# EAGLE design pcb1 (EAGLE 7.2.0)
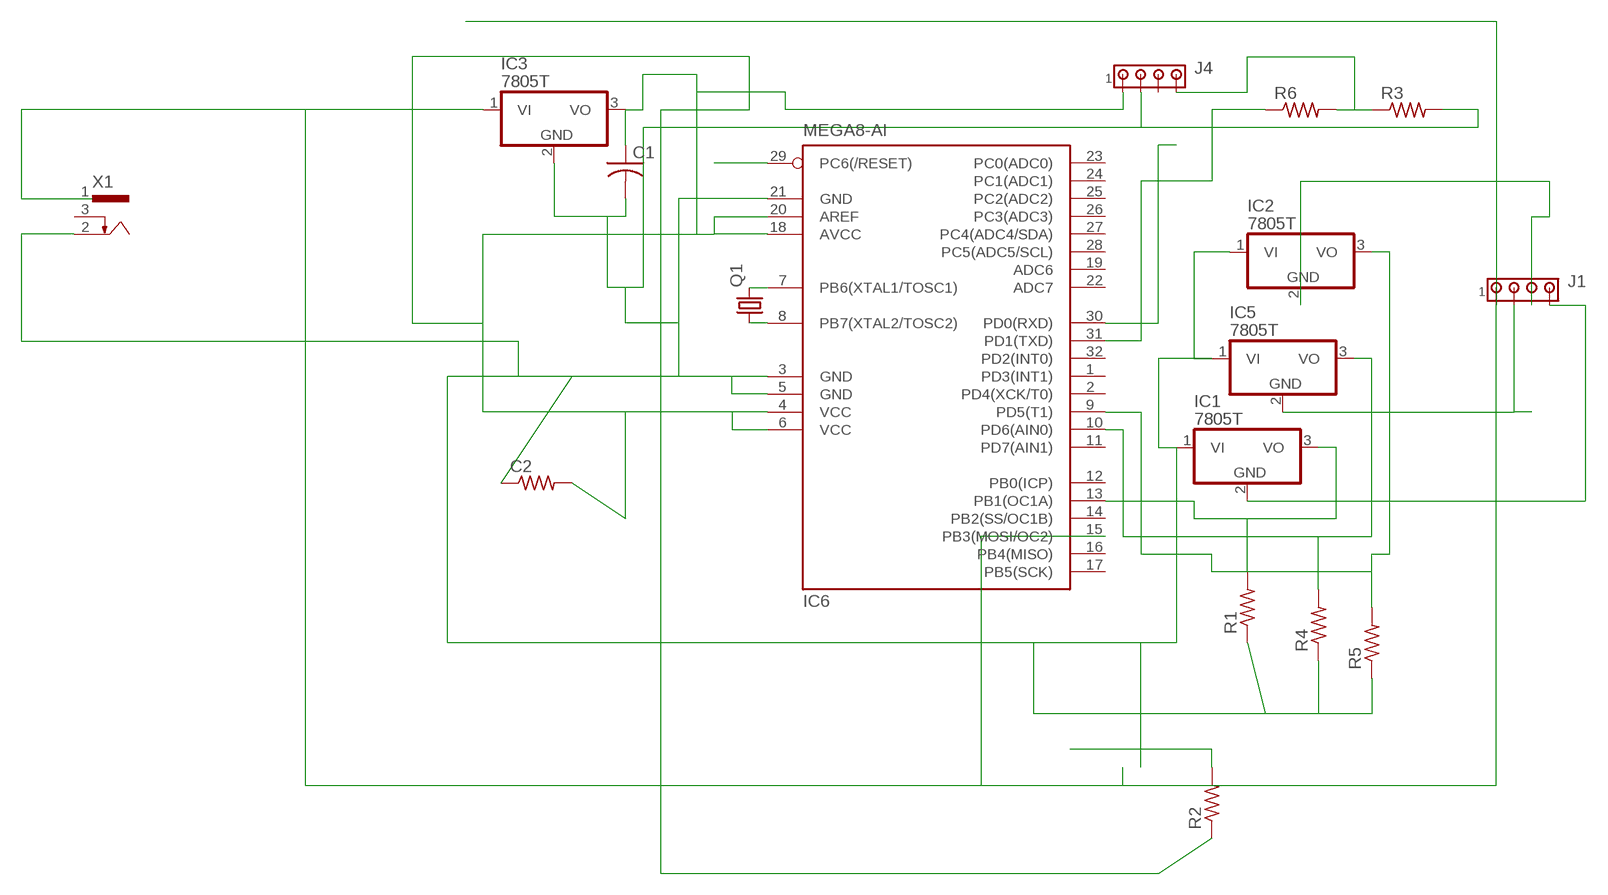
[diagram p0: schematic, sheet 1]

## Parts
C1  C-US025-025X050  [C025-025X050]
C2  R-US_M1206  [M1206]
IC1  7805T  [TO220H]
IC2  7805T  [TO220H]
IC3  7805T  [TO220H]
IC5  7805T  [TO220H]
IC6  MEGA8-AI  [TQFP32-08]
J1  MTA04-100  [10X04MTA]
J4  MTA04-100  [10X04MTA]
Q1  CRYSTALHC49S  [HC49/S]
R1  R-US_M1206  [M1206]
R2  R-US_M1206  [M1206]
R3  R-US_M1206  [M1206]
R4  R-US_M1206  [M1206]
R5  R-US_M1206  [M1206]
R6  R-US_M1206  [M1206]
X1  733980-62  [733980-62]

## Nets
N$1: IC6.7(PB6(XTAL1/TOSC1)) Q1.2
N$2: IC6.8(PB7(XTAL2/TOSC2)) Q1.1
N$5: IC2.2(GND) J1.3
N$6: IC1.3(VO) IC6.13(PB1(OC1A)) R1.2
N$7: IC6.15(PB3(MOSI/OC2))
N$8: IC5.3(VO) IC6.10(PD6(AIN0)) R4.2
N$9: R2.2
N$10: IC2.3(VO) IC6.9(PD5(T1)) R5.2
N$11: C1.2 C2.1 IC1.1(VI) IC2.1(VI) IC3.2(GND) IC5.1(VI) IC6.3(GND) IC6.5(GND) IC6.21(GND) J4.2 R1.1 R3.2 R4.1 R5.1 X1.2
N$12: IC5.2(GND) J1.2
N$13: IC1.2(GND) J1.4
N$14: IC6.29(PC6(/RESET))
N$15: IC6.30(PD0(RXD))
N$18: IC6.31(PD1(TXD)) R6.1
N$20: J4.4 R3.1 R6.2
N$23: IC3.1(VI) J1.1 X1.1
N$24: C1.1 C2.2 IC3.3(VO) IC6.4(VCC) IC6.6(VCC) IC6.18(AVCC) IC6.20(AREF) J4.1 R2.1
Unconnected: IC6.1(PD3(INT1)) IC6.2(PD4(XCK/T0)) IC6.11(PD7(AIN1)) IC6.12(PB0(ICP)) IC6.14(PB2(SS/OC1B)) IC6.16(PB4(MISO)) IC6.17(PB5(SCK)) IC6.19(ADC6) IC6.22(ADC7) IC6.23(PC0(ADC0)) IC6.24(PC1(ADC1)) IC6.25(PC2(ADC2)) IC6.26(PC3(ADC3)) IC6.27(PC4(ADC4/SDA)) IC6.28(PC5(ADC5/SCL)) IC6.32(PD2(INT0)) J4.3 X1.3

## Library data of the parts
C1 = adafruit:C-US: CAPACITOR, American symbol
C2 R1-R6 = adafruit:R-US_: RESISTOR, American symbol
IC1-IC3 IC5 = adafruit:78*: Positive VOLTAGE REGULATOR Added bigger pads to the TO-92 package
IC6 = atmel:MEGA8: MICROCONTROLLER 8 Kbytes FLASH, 1 kbytes SRAM, 512 bytes EEPROM, USART, 6-channel 10 bit ADC, 2-channel 8 bit ADC Pin compatible with Atmega48, ATMega88, ATMega168 Source: avr.lbr; MPN: ATMEGA8-16AU; OC_FARNELL: 9171371; OC_NEWARK: 73M8863
J1 J4 = con-amp:MTA04-100: AMP connector
Q1 = adafruit:CRYSTAL: CRYSTAL; OC_FARNELL: 1667008; OC_NEWARK: unknown
X1 = con-conrad:73398?: FEMALE PRINT CONNECTOR Niedervolt-Steckverbinder Distributor Conrad

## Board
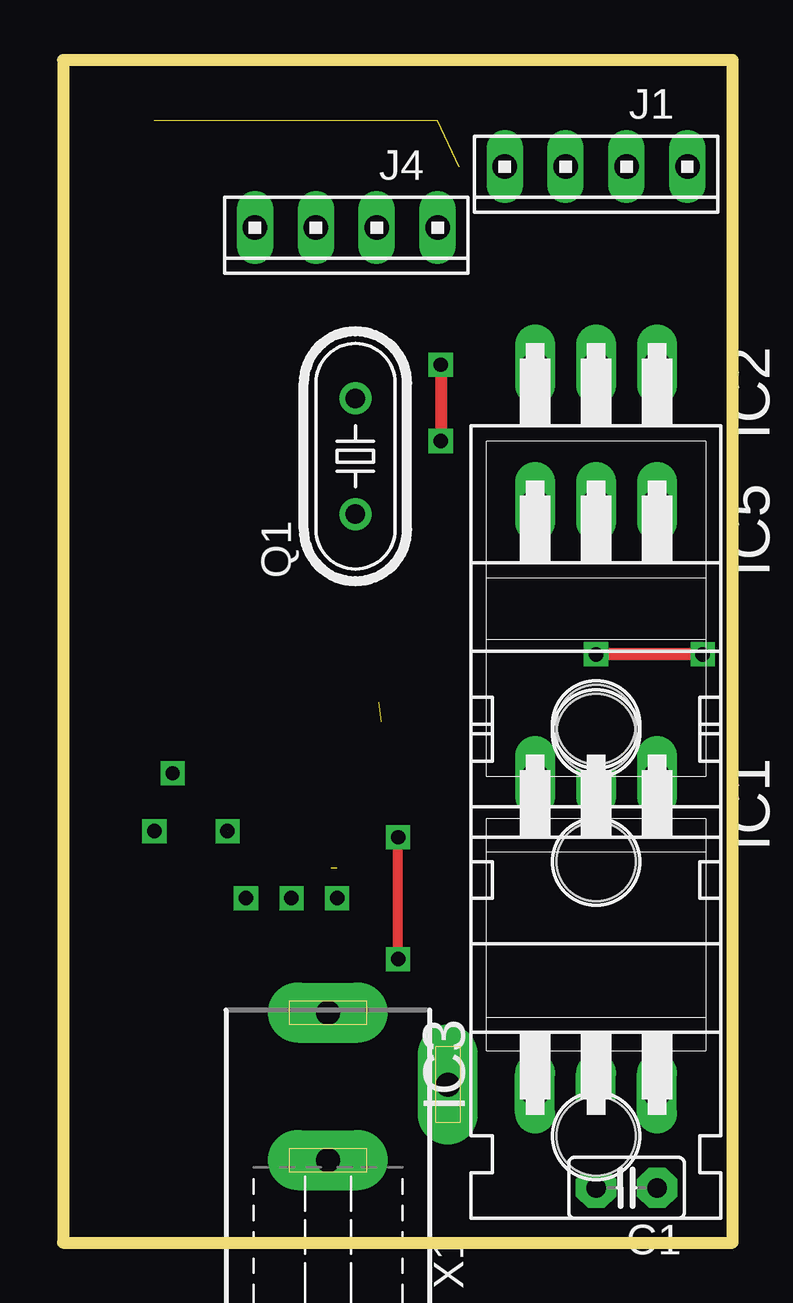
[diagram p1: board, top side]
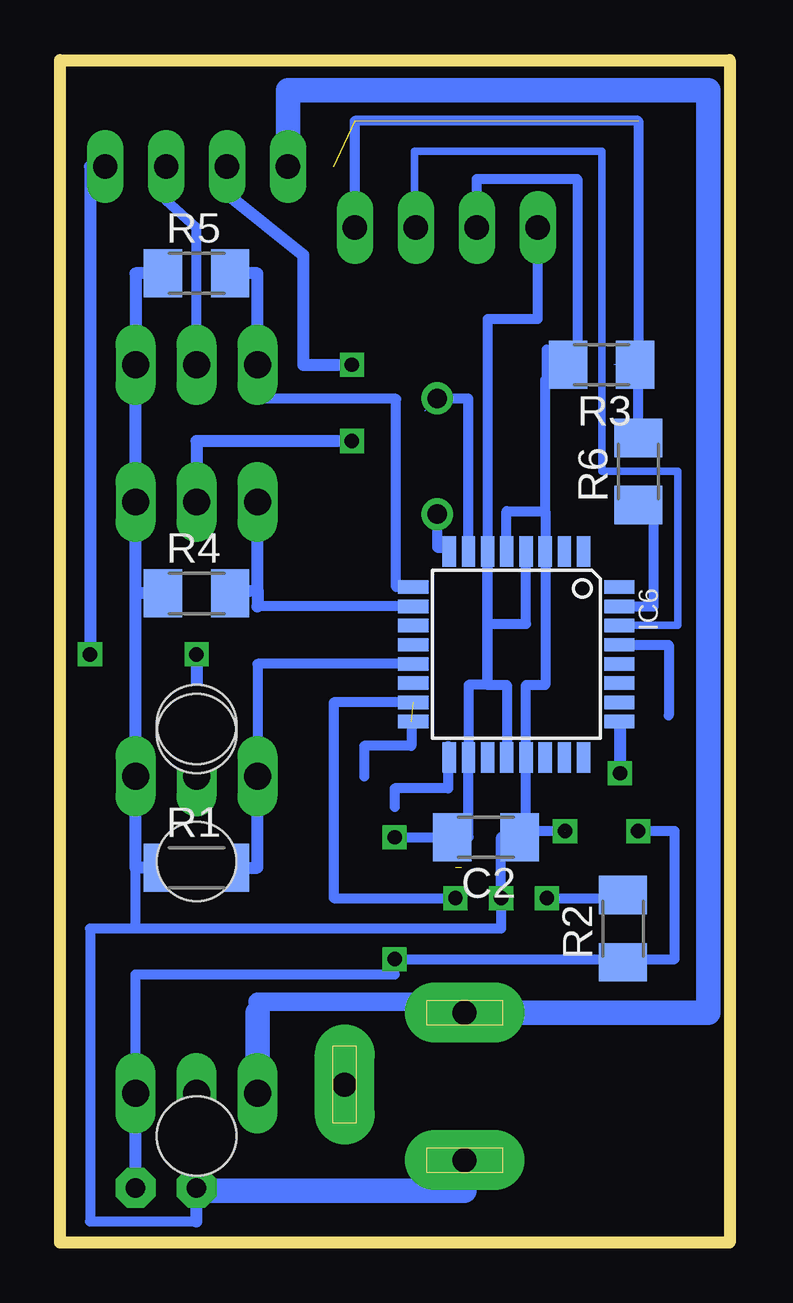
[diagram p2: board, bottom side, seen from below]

Size 27.92 x 49.28 mm. Coordinates in mm from the lower left corner, seen from the top.
Outline: 0,0 27.92,0 27.92,49.28 0,49.28 0,0
Copper layers (1*16): Top 0.035mm / dielectric 1.5mm / Bottom 0.035mm
Design rules "default": minimum track width 10mil, minimum drill 24mil, track to track 8mil, track to pad 8mil, pad to pad 8mil, via to via 8mil, smd to smd 8mil, copper to edge 40mil, drill to drill 8mil, minimum pad ring 10mil, minimum via ring 8mil, stop-mask expansion 4mil, vias tented up to drill 0mil, thermal gap 10mil

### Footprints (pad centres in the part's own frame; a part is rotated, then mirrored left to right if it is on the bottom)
C025-025X050 = drill 0.813 pad 1.676 octagon: 1 -1.27,0; 2 1.27,0
M1206 = smd 1.6 x 2: 1 -1.4,0; 2 1.4,0
TO220H = drill 1.118 long: 1 -2.54,-10.16; 2 0,-10.16; 3 2.54,-10.16 | hole 3.302: 0,4.826
TQFP32-08 = smd 1.27 x 0.559: 1 -4.293,2.8; 2 -4.293,2; 3 -4.293,1.2; 4 -4.293,0.4; 5 -4.293,-0.4; 6 -4.293,-1.2; 7 -4.293,-2; 8 -4.293,-2.8; 17 4.293,-2.8; 18 4.293,-2; 19 4.293,-1.2; 20 4.293,-0.4; 21 4.293,0.4; 22 4.293,1.2; 23 4.293,2; 24 4.293,2.8 | smd 0.559 x 1.27: 9 -2.8,-4.293; 10 -2,-4.293; 11 -1.2,-4.293; 12 -0.4,-4.293; 13 0.4,-4.293; 14 1.2,-4.293; 15 2,-4.293; 16 2.8,-4.293; 25 2.8,4.293; 26 2,4.293; 27 1.2,4.293; 28 0.4,4.293; 29 -0.4,4.293; 30 -1.2,4.293; 31 -2,4.293; 32 -2.8,4.293
10X04MTA = drill 1.016 long: 1 3.81,0; 2 1.27,0; 3 -1.27,0; 4 -3.81,0
HC49/S = drill 0.813: 1 -2.413,0; 2 2.413,0
733980-62 = drill 1 pad 2.5 long: 1 0,8.57; 2 0,2.42; 3 5,5.57

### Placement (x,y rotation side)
C1  23.5,2.29 180 top
C2  10.16,16.89 180 bottom
IC1  22.23,9.27 180 top
IC2  22.23,26.42 180 top
IC3  22.23,16.38 0 top
IC5  22.23,20.7 180 top
IC6  8.89,24.51 270 bottom
J1  22.23,44.83 180 top
J4  11.81,42.29 180 top
Q1  12.19,32.77 90 top
R1  22.23,15.62 0 bottom
R2  4.45,13.08 90 bottom
R3  5.33,36.58 180 bottom
R4  22.23,27.05 0 bottom
R5  22.23,40.39 0 bottom
R6  3.81,32.13 90 bottom
X1  11.05,1.02 0 top

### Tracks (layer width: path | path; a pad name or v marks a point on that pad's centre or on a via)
N$1
  Bottom 0: 12.7,34.67 Q1.2
  Bottom 0.406: IC6.7 10.89,35.18 Q1.2
N$2
  Bottom 0.406: Q1.1 12.19,28.96 11.69,28.96 IC6.8
N$3  (via drill 0.6)  (1 unrouted)
  other vias: 4.57,19.56 6.86,17.14
N$4  (via drill 0.6)
  other vias: 4.57,19.56
N$5
  Bottom 0.406: IC2.2 22.23,42.29 23.5,43.43 J1.3
N$6
  Bottom 0.406: IC6.13 19.69,24.11 IC1.3
  Bottom 0.508: R1.2 19.69,15.62 IC1.3
N$7  (1 unrouted)
  Bottom 0.406: IC6.15 16.51,22.51 16.51,14.35 11.43,14.35 | 13.27,21.71 13.27,20.7 15.24,20.7 15.24,19.43
N$8
  Bottom 0.406: IC6.10 19.69,26.51
  Bottom 0.508: 20.8,27.05 19.69,27.2 | R4.2 19.69,27.2 | 19.69,27.2 19.69,26.51 | 19.69,27.2 IC5.3
N$10
  Bottom 0.406: IC6.9 13.9,27.31 13.9,35.16 19.69,35.16 IC2.3
  Bottom 0.508: R5.2 19.69,40.39 IC2.3
N$11  (via drill 0.6)
  Bottom 0.406: 7.69,30.48 9.3,30.48 IC6.5 | 7.69,30.48 IC6.3 7.69,23.24 8.49,23.24 IC6.21 8.49,16.89 C2.1 9.53,16.89 v9.53,14.35 9.53,13.08 24.77,13.08 | 24.77,13.08 24.77,15.62 | 24.77,13.08 26.67,13.08 26.67,0.89 22.23,0.89 | 22.23,2.16 C1.2 | 7.69,30.48 7.69,35.94 R3.2 | 7.62,37.21 R3.2 | R3.2 7.62,35.94 7.62,37.21 | 7.62,37.21 6.35,37.21 6.35,44.32 10.54,44.32 J4.2 10.54,42.04
  Bottom 0.508: R1.1 24.77,15.62 IC1.1 24.77,27.05 | R4.1 24.77,27.05 | 24.77,27.05 IC5.1 IC2.1 24.77,40.39 R5.1 | IC3.2 C1.2 | 22.23,0.89 22.23,2.16
  Bottom 1.016: X1.2 11.05,2.16 22.23,2.16
N$12  (via drill 0.6)
  Top 0.508: v15.75,36.58 v15.75,33.4
  Bottom 0.508: v15.75,36.58 17.78,36.58 17.78,41.15 20.96,43.69 J1.2 | v15.75,33.4 22.23,33.4 IC5.2
N$13  (via drill 0.6)
  Top 0.508: v26.67,24.51 v22.23,24.51
  Bottom 0.406: J1.4 26.67,44.83
  Bottom 0.508: 26.67,44.83 v26.67,24.51 | v22.23,24.51 IC1.2
N$14
  Bottom 0.406: IC6.29 2.54,24.91 2.54,21.97 | 7.62,14.35 4.45,14.35
N$15
  Bottom 0.305: IC6.30 2.16,25.72 2.16,32.13 5.33,32.13 5.33,45.47 13.14,45.47 13.14,42.29
  Bottom 0.406: IC6.30 | 13.14,42.29 13.08,42.29
N$16  (via drill 0.6)
  other vias: 4.57,19.56
N$17
  Bottom 0.406: 11.73,20.7 11.73,18.92 13.97,18.92 13.97,18.16
N$18
  Bottom 0.406: R6.1 3.18,30.86 3.18,26.5 IC6.31
N$19  (1 unrouted)
N$20  (3 unrouted)
  Bottom 0: R3.1 4.83,36.58
  Bottom 0.406: R6.2 3.81,35.94 3.94,35.94 R3.1 3.81,36.58 3.81,46.74 15.62,46.74 J4.4
N$21  (via drill 0.6)
  other vias: 3.81,17.14 7.62,14.35 11.43,14.35
N$22
  Bottom 0.406: 3.81,11.81 2.29,11.81 2.29,17.14 3.81,17.14
N$23
  Bottom 0.508: X1.1 11.43,9.59 11.43,10.03 | 19.69,10.03 19.69,9.59
  Bottom 0.762: 11.43,10.03 19.69,10.03 | 11.43,9.59
  Bottom 1.016: J1.1 18.41,48.01 0.89,48.01 0.89,9.59 11.43,9.59 | 19.69,9.59 IC3.1
N$24  (via drill 0.6)
  Top 0.406: v13.97,11.81 v13.97,16.89
  Bottom 0.406: 10.09,25.78 8.49,25.78 IC6.4 | IC6.18 10.89,16.89 | 10.09,23.24 9.29,23.24 IC6.20 | IC6.6 | 10.09,25.78 10.09,23.24 | IC6.18 10.88,16.89 10.89,16.89 | 10.09,23.24 IC6.6 | v13.97,16.89 C2.2 10.89,16.89 | IC6.6 10.09,38.48 8,38.48 J4.1 | IC6.6 10.09,25.78 | 10.09,23.24 10.88,23.24 IC6.18 | IC3.3 24.9,6.22 24.77,5.46 24.77,11.18 13.97,11.18 v13.97,11.81 5.08,11.81 5.08,11.68 R2.1
  Bottom 0.508: C1.1 24.77,5.46 IC3.3
N$25
  Bottom 0.406: 6.86,17.14 8.13,17.14
N$26
  Bottom 0.508: 4.57,21.59 4.57,19.56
